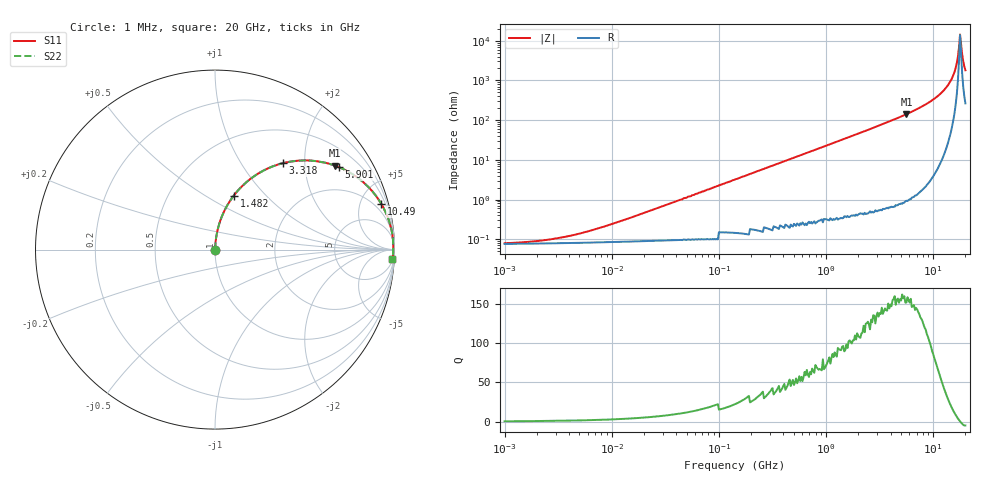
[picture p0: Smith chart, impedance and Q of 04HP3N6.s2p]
# MHz S MA R 50
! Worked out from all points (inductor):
!   431 points, 1 MHz to 20 GHz, reference 50 ohm
!   read as one part in series: L = 3.6 nH near 11.49 MHz
!   highest Q = 156 at 5.635 GHz (marker M1), where L = 4 nH
!   self-resonance near 17.82 GHz
!   S11 on the Smith chart (normalised r, x): 1 MHz: 1.00, +0.00; 1.482 GHz: 1.01, +0.68; 3.318 GHz: 1.01, +1.56; 5.901 GHz: 1.02, +2.99; 10.49 GHz: 1.09, +7.24; 20 GHz: 7, -35
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1  0.0005769 23.1  0.999 -0.0  0.999 -0.0  0.0005769 23.1
2.345  0.0007811 42.7  0.999 -0.0  0.999 -0.0  0.0007811 42.7
5.25  0.001346 61.8  0.999 -0.1  0.999 -0.1  0.001346 61.8
27.564  0.00629 81.7  0.999 -0.4  0.999 -0.4  0.00629 81.7
144.716  0.033 85.6  0.998 -1.9  0.998 -1.9  0.033 85.6
742.485  0.165 79.6  0.984 -9.5  0.984 -9.5  0.165 79.6
1481.697  0.319 70.8  0.944 -18.6  0.944 -18.6  0.319 70.8
3317.746  0.612 51.9  0.787 -37.7  0.787 -37.7  0.612 51.9
3898.162  0.677 47.0  0.731 -42.6  0.731 -42.6  0.677 47.0
5635.056  0.814 35.1  0.575 -54.5  0.575 -54.5  0.814 35.1
5900.693  0.829 33.6  0.554 -56.0  0.554 -56.0  0.829 33.6
10494.53  0.961 15.4  0.265 -73.9  0.265 -73.9  0.961 15.4
12911.73  0.983 9.3  0.161 -79.2  0.161 -79.2  0.983 9.3
14825.14  0.991 5.3  0.093 -81.6  0.093 -81.6  0.991 5.3
15885.69  0.993 3.3  0.059 -81.2  0.059 -81.2  0.993 3.3
16634.54  0.993 2.0  0.036 -78.4  0.036 -78.4  0.993 2.0
17418.69  0.993 0.7  0.015 -63.0  0.015 -63.0  0.993 0.7
17824.53  0.993 0.1  0.006919 -14.8  0.006919 -14.8  0.993 0.1
18239.81  0.993 -0.5  0.012 53.3  0.012 53.3  0.993 -0.5
18664.78  0.993 -1.2  0.022 69.7  0.022 69.7  0.993 -1.2
19544.64  0.991 -2.5  0.044 77.3  0.044 77.3  0.991 -2.5
20000  0.99 -3.1  0.055 78.4  0.055 78.4  0.99 -3.1
